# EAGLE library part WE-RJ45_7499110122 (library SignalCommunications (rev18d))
Order Code 7499110122 Design THT xBase-T 10/100/1000 Base-T Ports 1x1 Application Standard Tab Position Down LED (Left-Right) YELLOW-GREEN EMI Fingers No Details see: http://katalog.we-online.de/en/pbs/WE-LAN_RJ45/7499110122? Updated by Yingchun Shan 2016-08-29 2016(C) Würth Elektronik
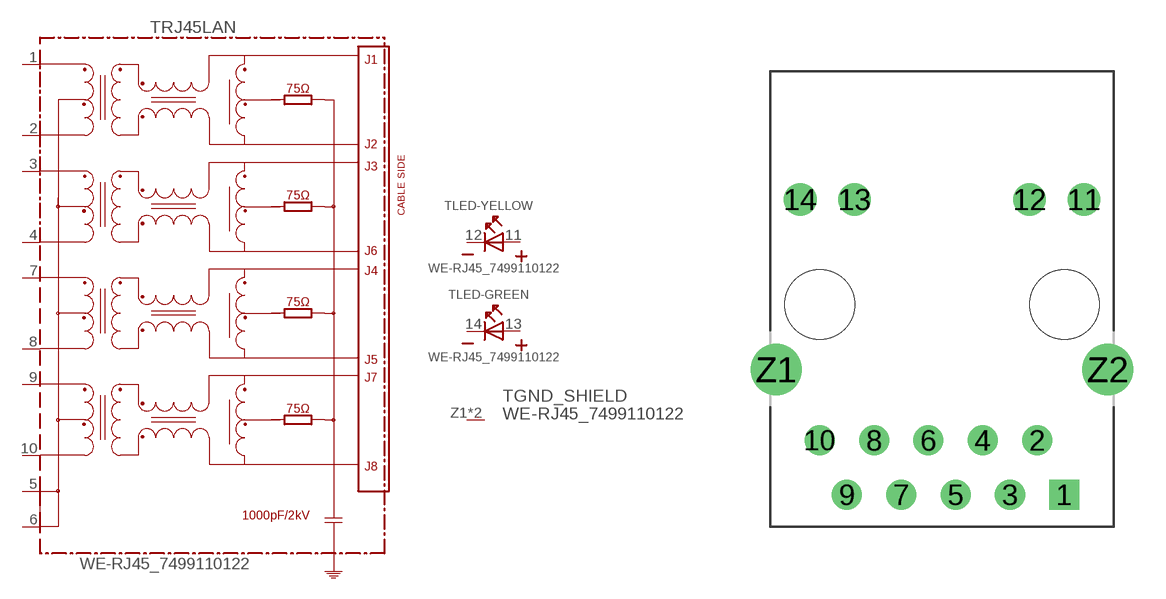
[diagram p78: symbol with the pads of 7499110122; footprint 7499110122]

Designator prefix T; gates RJ45LAN=7499110122 LED-YELLOW=LED2PIN LED-GREEN=LED2PIN GND_SHIELD=GNDPIN

## WE-RJ45_7499110122 (COMPANY-URL: http://www.we-online.de; CREATED-BY: Christin Zierenner; CREATED-DATE: AUG 2012; DATASHEET-URL: http://katalog.we-online.de/kataloge/eisos/media/pdf/7499110122.pdf; MANUFACTURER: Würth Elektronik eiSos GmbH)  [7499110122]
1  RJ45LAN:1
2  RJ45LAN:2
3  RJ45LAN:3
4  RJ45LAN:4
5  RJ45LAN:5
6  RJ45LAN:6
7  RJ45LAN:7
8  RJ45LAN:8
9  RJ45LAN:9
10  RJ45LAN:10
11  LED-YELLOW:A  pas
12  LED-YELLOW:K  pas
13  LED-GREEN:A  pas
14  LED-GREEN:K  pas
Z1  GND_SHIELD:GND  pwr
Z2  GND_SHIELD:GND  pwr

## Footprint 7499110122 (pad centres in mm)
MAX HEIGHT=13.50mm PORTS----1X1 LED -YES
drill 0.9 square: 1 5.715,-8.89
drill 0.9: 2 4.445,-6.35; 3 3.175,-8.89; 4 1.905,-6.35; 5 0.635,-8.89; 6 -0.635,-6.35; 7 -1.905,-8.89; 8 -3.175,-6.35; 9 -4.445,-8.89; 10 -5.715,-6.35
drill 1.02: 11 6.63,4.9; 12 4.09,4.9; 13 -4.09,4.9; 14 -6.63,4.9
drill 1.6: Z1 -7.745,-3.05; Z2 7.745,-3.05
hole 3.25 at 5.715,0
hole 3.25 at -5.715,0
